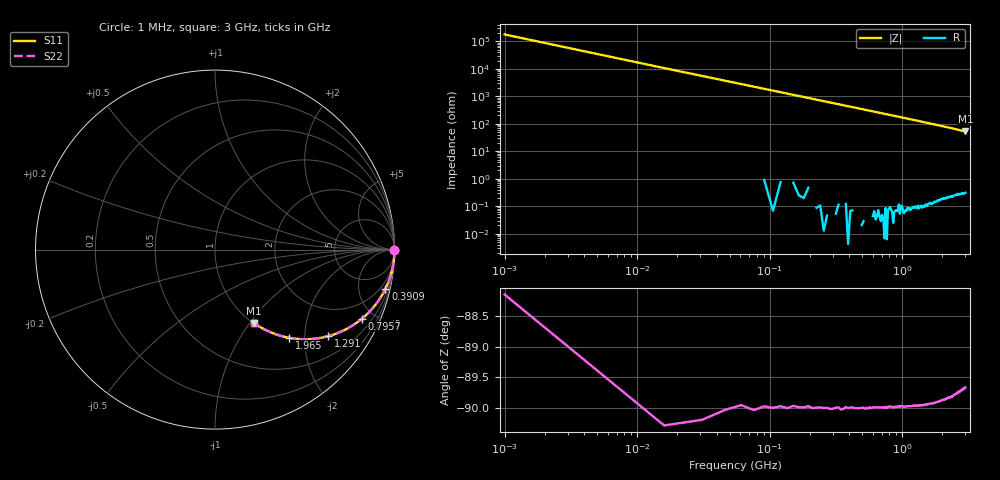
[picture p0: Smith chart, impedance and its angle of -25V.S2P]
!Keysight Technologies,E4991B,MY54301043,A.02.04
!Date: Thu Nov 16 21:17:16 2023
!Data:
!Freq	S11	S21	S12	S22
# Hz S MA R 50
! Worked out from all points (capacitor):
!   201 points, 1 MHz to 3 GHz, reference 50 ohm
!   read as one part in series: C = 936 fF near 15.99 MHz
!   lowest |Z| = 52.3 ohm at 3 GHz (marker M1)
!   S11 on the Smith chart (normalised r, x): 1 MHz: open; 390.9 MHz: 1.00, -8.69; 795.7 MHz: 1.00, -4.25; 1.291 GHz: 1.00, -2.61; 1.965 GHz: 1.00, -1.68; 3 GHz: 1.01, -1.05
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1000000  1 -0.0  0.000565 88.1  0.000565 88.1  1 -0.0
1.5995e7  1 -0.5  0.009436 89.7  0.009436 89.7  1 -0.5
3.099e7  0.9999 -1.0  0.01821 89.1  0.01821 89.1  0.9999 -1.0
4.5985e7  0.9996 -1.5  0.02704 88.5  0.02704 88.5  0.9996 -1.5
6.098e7  0.9993 -2.1  0.03584 87.9  0.03584 87.9  0.9993 -2.1
7.5975e7  0.999 -2.6  0.04464 87.5  0.04464 87.5  0.999 -2.6
1.05965e8  0.9981 -3.6  0.06223 86.4  0.06223 86.4  0.9981 -3.6
1.35955e8  0.9968 -4.6  0.07979 85.4  0.07979 85.4  0.9968 -4.6
1.8094e8  0.9944 -6.1  0.1059 83.9  0.1059 83.9  0.9944 -6.1
2.25925e8  0.9913 -7.6  0.1318 82.4  0.1318 82.4  0.9913 -7.6
2.7091e8  0.9875 -9.1  0.1574 80.9  0.1574 80.9  0.9875 -9.1
3.9087e8  0.9745 -13.0  0.2243 77.0  0.2243 77.0  0.9745 -13.0
5.1083e8  0.9575 -16.8  0.2882 73.2  0.2882 73.2  0.9575 -16.8
6.3079e8  0.9372 -20.4  0.3488 69.6  0.3488 69.6  0.9372 -20.4
7.95735e8  0.9049 -25.2  0.4254 64.8  0.4254 64.8  0.9049 -25.2
1.005665e9  0.859 -30.8  0.5115 59.2  0.5115 59.2  0.859 -30.8
1.29057e9  0.793 -37.5  0.6088 52.5  0.6088 52.5  0.793 -37.5
1.5005e9  0.7443 -41.8  0.6671 48.1  0.6671 48.1  0.7443 -41.8
1.965345e9  0.6431 -49.9  0.7644 40.0  0.7644 40.0  0.6431 -49.9
2.01033e9  0.6339 -50.5  0.772 39.3  0.772 39.3  0.6339 -50.5
2.505165e9  0.5412 -57.0  0.8388 32.8  0.8388 32.8  0.5412 -57.0
3e9  0.4623 -62.1  0.884 27.5  0.884 27.5  0.4623 -62.1
